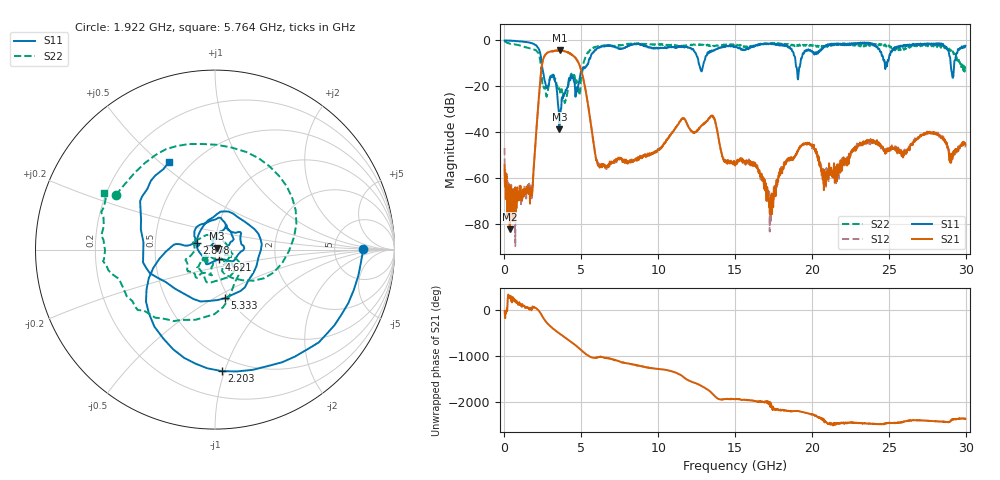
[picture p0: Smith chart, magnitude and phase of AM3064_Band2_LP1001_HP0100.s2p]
# Hz S DB R 50.0
!freq dBS11 angS11 dBS21 angS21 dBS12 angS12 dBS22 angS22
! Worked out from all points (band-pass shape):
!   1600 points, 10 MHz to 29.98 GHz, reference 50 ohm
!   highest |S21| = -4.32 dB at 3.59 GHz (marker M1); lowest = -82.3 dB at 347.4 MHz (marker M2)
!   |S21| within 3 dB of the highest: 2.567 GHz to 4.575 GHz (2.008 GHz wide, 56.2 % of centre)
!   lowest |S11| = -38.8 dB at 3.571 GHz (marker M3), VSWR 1.02, Z = 50.9 + j0.744 ohm
!   |S11| at or under -10 dB: 2.427 GHz to 5.451 GHz (3.024 GHz wide, 76.8 % of centre); 12.64 GHz to 12.95 GHz (313.3 MHz wide, 2.45 % of centre); 18.94 GHz to 19.25 GHz (305.5 MHz wide, 1.6 % of centre)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
!   |S22| runs from -27.3 to -0.2 dB; largest |S21 - S12| = 0.02
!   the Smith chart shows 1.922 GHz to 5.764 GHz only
!   S11 on the Smith chart (normalised r, x): 1.922 GHz: 11, +0; 2.203 GHz: 0.39, -0.98; 2.878 GHz: 0.82, +0.06; 4.621 GHz: 1.04, -0.11; 5.333 GHz: 0.95, -0.56; 5.764 GHz: 0.38, +0.54
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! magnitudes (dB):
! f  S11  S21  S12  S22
! 10 MHz  0.0  -54.4  -46.9  -0.2
! 347.4 MHz  -0.1  -82.3  -76.3  -1.3
! 1.697 GHz  -1.1  -65.7  -62.7  -3.6
! 1.922 GHz  -1.7  -53.7  -53.9  -4.0
! 2.203 GHz  -3.4  -27.9  -27.8  -5.5
! 2.878 GHz  -19.5  -5.1  -5.1  -19.3
! 3.571 GHz  -38.8  -4.4  -4.4  -20.9
! 3.59 GHz  -35.3  -4.3  -4.5  -21.5
! 4.621 GHz  -24.6  -7.6  -7.6  -18.9
! 5.015 GHz  -13.0  -13.6  -13.6  -14.8
! 5.333 GHz  -11.2  -23.9  -23.8  -6.3
! 5.764 GHz  -5.2  -43.2  -43.5  -3.2
! 6.214 GHz  -3.0  -55.2  -54.7  -2.4
! 10 GHz  -3.4  -47.7  -47.7  -1.8
! 13.49 GHz  -4.4  -32.9  -32.9  -2.2
! 15 GHz  -2.6  -54.6  -53.3  -1.9
! 17.35 GHz  -1.4  -70.8  -71.4  -1.2
! 18.29 GHz  -2.3  -53.4  -52.9  -2.0
! 19.99 GHz  -4.5  -46.2  -45.8  -2.0
! 20.78 GHz  -2.8  -65.3  -61.0  -2.9
! 25 GHz  -8.2  -47.1  -47.5  -2.2
! 29.98 GHz  -2.3  -45.5  -46.7  -10.9
